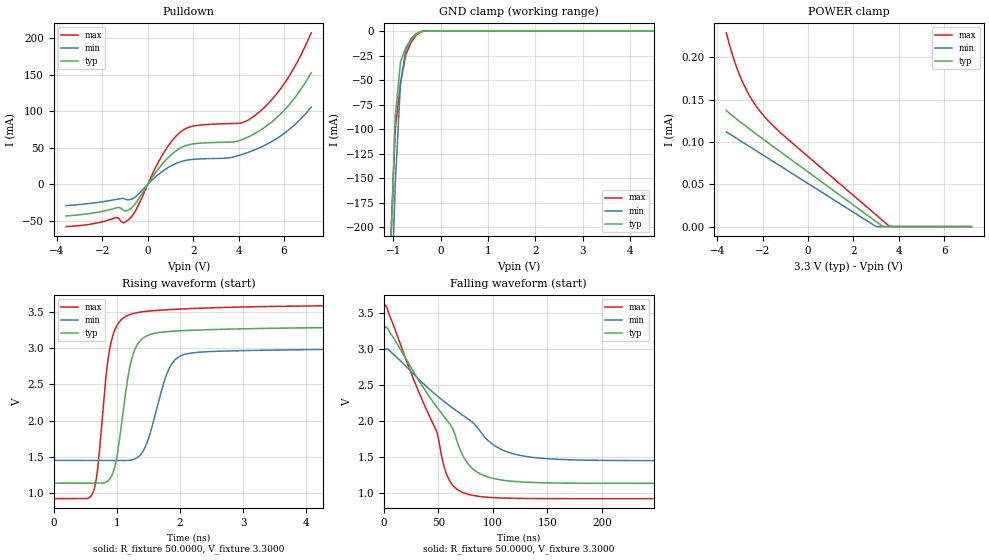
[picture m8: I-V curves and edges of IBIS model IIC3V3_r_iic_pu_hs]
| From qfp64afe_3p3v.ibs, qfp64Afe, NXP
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[Model] IIC3V3_r_iic_pu_hs
|   Model IIC3V3_r_iic_pu_hs
| This model was characterised for following simulation conditions:
| External (pad) voltage:
|   - Typ: 3.3V,   - Min: 3.0V,   - Max: 3.6V
| Library cells for typ/min/max conditions are connected as defined below:
|  IO - External Pad
|  A - Core Input
|  EN - Output Buffer Enable
|  BOOST - vdde
|  ECS - vdd
|  EGP - gnd
|  ENZI - vdd
|  EPD - vdd
|  EPUN - gnd
|  SSEL - vdd
|  ZI - NC
|  ZIF - NC
|  gnd - gnd
|  gnde - gnde
|  vdd - vdd
|  vdde - vdde
| All other pins connected to ground
Model_type I/O_open_drain
Polarity   Non-Inverting
Enable   Active-Low
Vinl =   0.9900V
Vinh =   2.3100V
Vmeas =  1.6500V
Cref =   0.0F
Rref =   1.0000k
Vref =   3.3000V
C_comp   3.5907pF   3.4406pF   3.7387pF
|C_comp_pullup   0.9138pF   0.8999pF   0.9173pF
|C_comp_pulldown   2.3268pF   2.4803pF   2.1806pF
[Model Spec]
| variable   typ   min   max
Vinh   0.9900V   0.9000V   1.0800V
Vinl   2.3100V   2.1000V   2.5200V
Vmeas   1.6500V   1.5000V   1.8000V
Vref   3.3000V   3.0000V   3.6000V
Cref   0.0F   0.0F   0.0F
Rref   1.0000k   1.0000k   1.0000k
[Temperature Range]   25.0000   0.1250k   -40.0000
[Voltage Range]   3.3000V   3.0000V   3.6000V
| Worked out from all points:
|   slope of the pulldown table from 0 to 0.495 V, typ, clamps not added: 22 ohm
|   GND clamp passes 1 mA (typ) near -0.43 V on its own axis
|   rising waveform, R_fixture 50.0000, V_fixture 3.3000: 20-80 % time 227ps typ, 309ps min, 192ps max; typ from 1.14 V to 3.3 V
|   falling waveform, R_fixture 50.0000, V_fixture 3.3000: 20-80 % time 50.8ns typ, 68.6ns min, 38.5ns max; typ from 3.3 V to 1.14 V
[Pulldown]
|Voltage   I(typ)   I(min)   I(max)
-3.6V     -43.22mA   -29.09mA   -57.9mA
-1.29V    -31.46mA   -20.15mA   -46.47mA
-1.07V    -35.79mA   -19.19mA   -52.9mA
-850mV    -35.14mA   -21.36mA   -48.43mA
-520mV    -25.35mA   -16.52mA   -35.11mA
580mV     25.81mA    16.3mA     36.8mA
1.24V     45.79mA    28.53mA    65.82mA
1.9V      54.89mA    33.9mA     79.08mA
4.1V      60.55mA    40.38mA    84.05mA
4.76V     70.44mA    47.87mA    95.32mA
6.08V     103.9mA    71.39mA    141.2mA
7.2V      152.9mA    106mA      207.6mA
[GND_clamp]
|Voltage   I(typ)   I(min)   I(max)
-3.6V     -5.602A    -5.487A    -5.717A
-1.07V    -242mA     -316.8mA   -230.5mA
-960mV    -86.76mA   -154.7mA   -99.49mA
-850mV    -31.82mA   -53.09mA   -53.51mA
-740mV    -16.97mA   -19.87mA   -24.44mA
-630mV    -8.597mA   -7.926mA   -11.89mA
-520mV    -3.004mA   -2.733mA   -4.196mA
-410mV    -439.7uA   -501.8uA   -589.4uA
7.2V      0A         0A         0A
[POWER_clamp]
|Voltage   I(typ)   I(min)   I(max)
-3.6V     137uA      111.9uA    228.9uA
-3.47V    134.1uA    109.7uA    215.6uA
-3.25V    129.3uA    106uA      196.2uA
-2.92V    122.3uA    100.4uA    172.9uA
-2.48V    113.3uA    92.88uA    150.2uA
-2.04V    104.5uA    85.42uA    133.7uA
-1.16V    87.2uA     70.51uA    109.7uA
2.91V     7.626uA    1.527uA    15.86uA
3.02V     5.475uA    0A         13.33uA
3.24V     1.173uA    0A         8.273uA
3.57V     0A         0A         687.1nA
7.2V      0A         0A         0A
[Ramp]
| variable   typ   min   max
dV/dt_r  1.2983/0.2270n   0.9293/0.3087n   1.6062/0.1923n
dV/dt_f  1.2983/50.7615n   0.9293/68.6289n   1.6062/38.4613n
R_load = 50.0000
[Rising Waveform]
R_fixture= 50.0000
V_fixture= 3.3000
V_fixture_min= 3.0000
V_fixture_max= 3.6000
|time   V(typ)   V(min)   V(max)
0s        1.135V     1.45V      921.3mV
624.4ps   1.134V     1.45V      1.015V
887.3ps   1.194V     1.45V      3V
996.2ps   1.488V     1.449V     3.308V
1.148ns   2.452V     1.448V     3.444V
1.365ns   3.101V     1.52V      3.499V
1.809ns   3.23V      2.685V     3.532V
2.033ns   3.242V     2.902V     3.542V
5.424ns   3.291V     2.989V     3.591V
1us       3.299V     2.999V     3.598V
[Falling Waveform]
R_fixture= 50.0000
V_fixture= 3.3000
V_fixture_min= 3.0000
V_fixture_max= 3.6000
|time   V(typ)   V(min)   V(max)
0s        3.299V     2.999V     3.598V
2.499ns   3.299V     3.008V     3.588V
48.53ns   2.195V     2.354V     1.847V
54.47ns   2.076V     2.28V      1.409V
59.61ns   1.976V     2.219V     1.188V
73.83ns   1.48V      2.066V     998.9mV
83.1ns    1.316V     1.956V     962.3mV
110.9ns   1.174V     1.584V     929.1mV
163.6ns   1.138V     1.466V     921.8mV
1us       1.135V     1.45V      921.3mV
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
